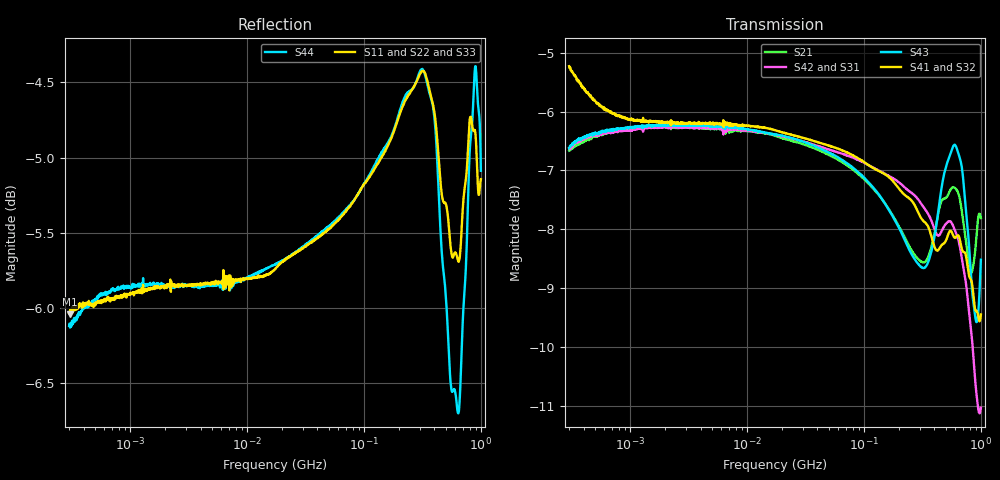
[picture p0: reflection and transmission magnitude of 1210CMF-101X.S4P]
!s-Parameter Generated by FASTRON Sdn. Bhd.
!FASTRON P/N : 1210CMF-101X
!Keysight Technologies: E5071C_MY46733604_B.14.02
!Date: Mon Mar 09 14:32:57 2026
!Version  :Rev00  Mon Mar 09 14:32:57 2026
!Data & Calibration Information:
!Freq	S11:SOLT4(ON)	S12:SOLT4(ON)	S13:SOLT4(ON)	S14:SOLT4(ON)
!	S21:SOLT4(ON)	S22:SOLT4(ON)	S23:SOLT4(ON)	S24:SOLT4(ON)
!	S31:SOLT4(ON)	S32:SOLT4(ON)	S33:SOLT4(ON)	S34:SOLT4(ON)
!	S41:SOLT4(ON)	S42:SOLT4(ON)	S43:SOLT4(ON)	S44:SOLT4(ON)
!PortZ  Port1:50+j0  Port2:50+j0  Port3:50+j0  Port4:50+j0
!When reading reference impedance value at option line is always used.
! Remarks : This data is being provided solely for informational purposes.
# Hz S dB R 50
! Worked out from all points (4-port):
!   1601 points, 300 kHz to 1 GHz, reference 50 ohm
!   strongest paths, dB at 300 kHz, 2.303 MHz, 17.55 MHz, 132.8 MHz, 1 GHz:
!     S41: -5.2, -6.2, -6.3, -7.0, -9.5
!     S32: -5.3, -6.2, -6.3, -7.0, -10.3
!     S43: -6.6, -6.2, -6.4, -7.4, -8.5
!     S42: -6.6, -6.3, -6.4, -7.0, -11.0
!     S31: -6.6, -6.3, -6.4, -7.0, -10.6
!     S21: -6.7, -6.3, -6.4, -7.4, -7.8
!   lowest |S11| = -6.0 dB at 303.6 kHz (marker M1), VSWR 2.99, Z = 135 + j41.6 ohm
!   |S11| at or under -10 dB: nowhere
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300000  -6.03 13.7  -6.69 16.0  -6.68 -164.1  -5.32 -14.1
        -6.66 15.7  -6.04 14.1  -5.27 -14.3  -6.72 -164.1
        -6.63 -164.5  -5.29 -14.1  -6.01 13.9  -6.72 16.0
        -5.23 -14.5  -6.62 -164.4  -6.62 15.6  -6.12 14.7
303584  -6.04 13.4  -6.67 15.7  -6.68 -164.2  -5.35 -14.0
        -6.66 15.6  -6.02 13.7  -5.30 -14.3  -6.73 -164.4
        -6.64 -164.3  -5.29 -14.2  -6.03 13.6  -6.69 15.9
        -5.25 -14.3  -6.62 -164.6  -6.60 15.4  -6.11 14.5
3897463  -5.84 1.5  -6.26 0.5  -6.24 179.6  -6.18 -3.0
         -6.27 0.6  -5.84 1.5  -6.18 -2.9  -6.28 179.5
         -6.28 179.5  -6.20 -3.0  -5.82 1.5  -6.26 0.5
         -6.19 -3.0  -6.29 179.6  -6.23 0.6  -5.85 1.5
5.743291e7  -5.43 1.6  -6.79 -4.2  -6.64 160.7  -6.62 -19.1
            -6.80 -4.2  -5.41 0.9  -6.63 -19.5  -6.69 160.4
            -6.66 160.6  -6.65 -19.6  -5.38 1.3  -6.79 -4.1
            -6.61 -19.2  -6.68 160.3  -6.76 -4.1  -5.41 1.3
2.925348e8  -4.47 -5.6  -8.50 -0.3  -7.61 92.5  -7.73 -86.8
            -8.51 -0.4  -4.46 -7.4  -7.83 -88.0  -7.51 91.9
            -7.64 92.6  -7.85 -87.9  -4.34 -6.3  -8.61 0.7
            -7.72 -86.8  -7.50 91.9  -8.59 0.8  -4.45 -6.5
6.162404e8  -5.64 -2.1  -7.32 1.3  -8.46 4.4  -8.16 -176.1
            -7.32 1.4  -5.80 -4.2  -8.54 -179.8  -8.09 6.2
            -8.47 4.5  -8.55 -179.8  -6.21 -5.9  -6.59 2.0
            -8.13 -176.0  -8.08 6.2  -6.61 2.1  -6.62 -1.8
1e9  -5.14 7.9  -7.79 4.0  -10.65 -100.7  -9.45 87.8
     -7.81 4.2  -6.39 10.3  -10.28 80.1  -11.07 -90.6
     -10.63 -100.7  -10.26 79.8  -4.98 -0.4  -8.57 19.1
     -9.45 87.7  -11.03 -90.7  -8.52 19.4  -5.09 -1.6
